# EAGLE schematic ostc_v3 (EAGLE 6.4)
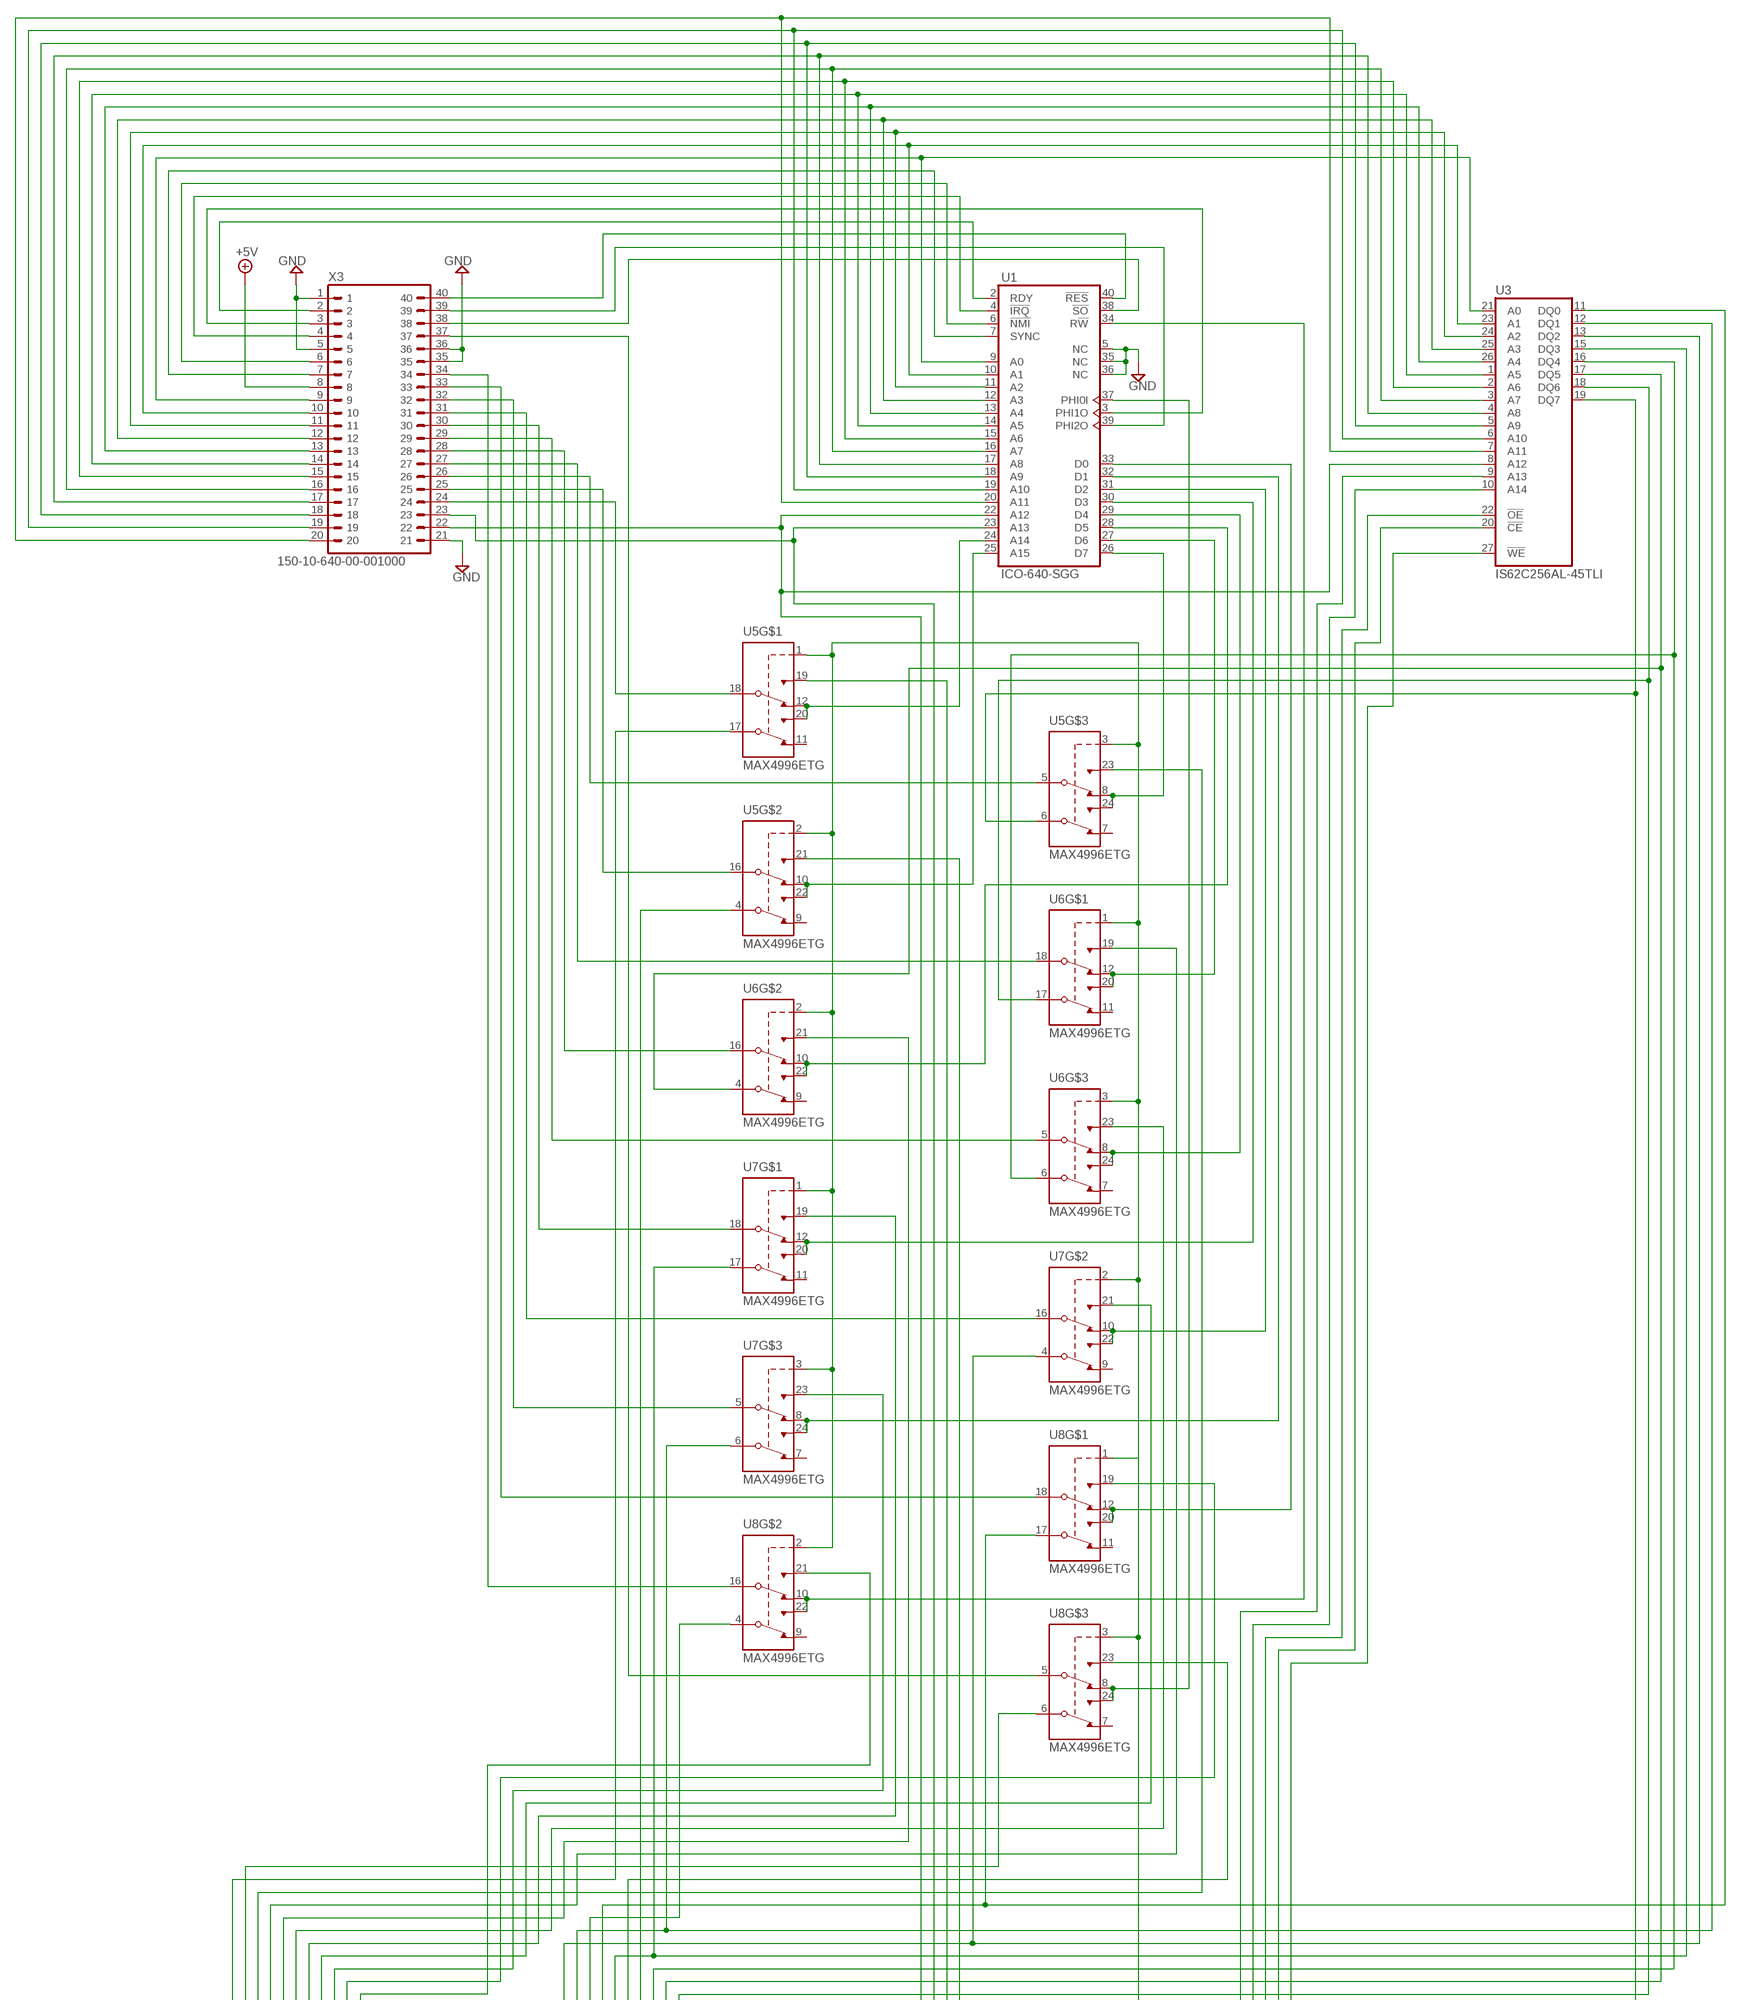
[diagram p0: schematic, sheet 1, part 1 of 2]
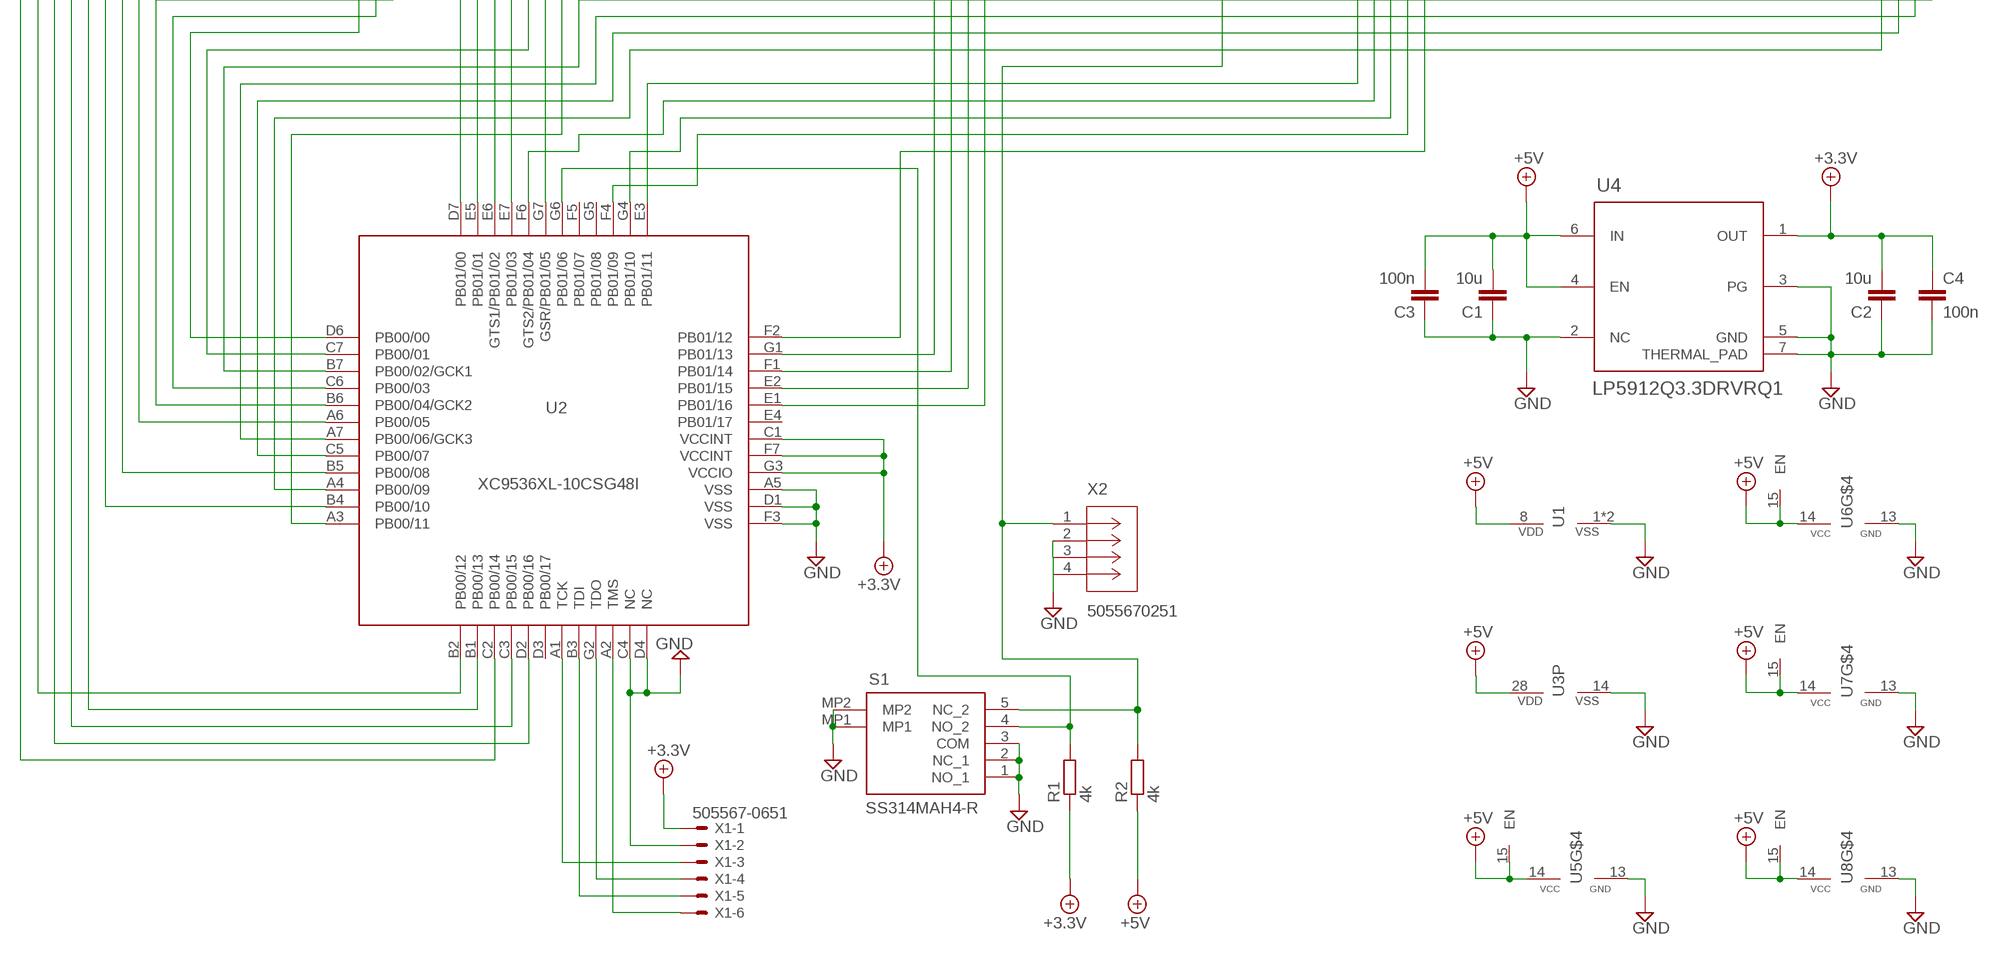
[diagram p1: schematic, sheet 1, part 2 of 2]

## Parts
C1  10u  C-EUC1206K  [C1206K]
C2  10u  C-EUC1206K  [C1206K]
C3  100n  C-EUC1206K  [C1206K]
C4  100n  C-EUC1206K  [C1206K]
R1  4k  R-EU_R0805  [R0805]
R2  4k  R-EU_R0805  [R0805]
S1  SS314MAH4-R  [SS314MAH4R]
U1  ICO-640-SGG  6502  [DIL40_LOWPROFILE]
U2  XC9536XL-10CSG48I  CX9536_CS48  [CSBGA48]
U3  IS62C256AL-45TLI  CY62256LL-ZC  [TSOP1-28]
U4  LP5912Q3.3DRVRQ1  LP5912-3.0DRVT  [DRV0006A-IPC_A]
U5  MAX4996ETG  [TQFN24]
U6  MAX4996ETG  [TQFN24]
U7  MAX4996ETG  [TQFN24]
U8  MAX4996ETG  [TQFN24]
X1  505567-0651  53261-06  [53261-06]
X2  5055670251  [CON_5055670251]
X3  150-10-640-00-001000  DIL40  [DIL40]

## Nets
+3.3V: C2.2 C4.1 R1.1 U2.C1(VCCINT) U2.F7(VCCINT) U2.G3(VCCIO) U4.1(OUT) X1.1
+5V: C1.2 C3.2 R2.1 U1.8(VDD) U3.28(VDD) U4.4(EN) U4.6(IN) U5.14(VCC) U5.15(EN) U6.14(VCC) U6.15(EN) U7.14(VCC) U7.15(EN) U8.14(VCC) U8.15(EN) X3.8
GND: C1.1 C2.1 C3.1 C4.2 S1.1(NO_1) S1.2(NC_1) S1.3(COM) S1.MP1 S1.MP2 U1.1(VSS) U1.5(NC) U1.21(VSS) U1.35(NC) U1.36(NC) U2.A5(VSS) U2.C4(NC) U2.D1(VSS) U2.D4(NC) U2.F3(VSS) U3.14(VSS) U4.2(NC) U4.3(PG) U4.5(GND) U4.7(THERMAL_PAD) U5.13(GND) U6.13(GND) U7.13(GND) U8.13(GND) X1.2 X2.2 X2.3 X2.4 X3.1 X3.5 X3.21 X3.35 X3.36
N$1: U1.2(RDY) X3.2
N$2: U1.3(PHI1O) X3.3
N$3: U1.4(!IRQ) X3.4
N$4: U1.6(!NMI) X3.6
N$5: U1.7(SYNC) X3.7
N$6: U1.9(A0) U3.21(A0) X3.9
N$7: U1.10(A1) U3.23(A1) X3.10
N$8: U1.11(A2) U3.24(A2) X3.11
N$9: U1.12(A3) U3.25(A3) X3.12
N$10: U1.13(A4) U3.26(A4) X3.13
N$11: U1.14(A5) U3.1(A5) X3.14
N$12: U1.15(A6) U3.2(A6) X3.15
N$13: U1.16(A7) U3.3(A7) X3.16
N$14: U1.17(A8) U3.4(A8) X3.17
N$15: U1.18(A9) U3.5(A9) X3.18
N$16: U1.19(A10) U3.6(A10) X3.19
N$17: U1.20(A11) U3.7(A11) X3.20
N$18: U2.E2(PB01/15) U5.19(NO1)
N$19: U1.22(A12) U2.G1(PB01/13) U3.8(A12) X3.22
N$20: U1.23(A13) U2.F1(PB01/14) X3.23
N$21: U2.E1(PB01/16) U5.21(NO1)
N$22: U2.D2(PB00/16) U5.23(NO1)
N$23: U2.C3(PB00/15) U6.19(NO1)
N$24: U2.B1(PB00/13) U6.21(NO1)
N$25: U2.B4(PB00/10) U6.23(NO1)
N$26: U2.B5(PB00/08) U7.19(NO1)
N$27: U2.A6(PB00/05) U7.21(NO1)
N$28: U2.B6(PB00/04/GCK2) U7.23(NO1)
N$29: U2.C6(PB00/03) U8.19(NO1)
N$30: U2.D6(PB00/00) U8.21(NO1)
N$31: U8.5(COM1) X3.37
N$32: U1.38(!SO) X3.38
N$33: U1.39(PHI2O) X3.39
N$34: U1.40(!RES) X3.40
N$35: U2.B2(PB00/12) U8.6(COM2)
N$36: U2.E6(GTS1/PB01/02) U8.4(COM2)
N$37: U2.E7(PB01/03) U3.11(DQ0) U8.17(COM2)
N$38: U2.E5(PB01/01) U3.12(DQ1) U7.6(COM2)
N$39: U2.D7(PB01/00) U3.13(DQ2) U7.4(COM2)
N$40: U2.C7(PB00/01) U3.15(DQ3) U7.17(COM2)
N$41: U2.B7(PB00/02/GCK1) U3.16(DQ4) U6.6(COM2)
N$42: U2.A7(PB00/06/GCK3) U3.17(DQ5) U6.4(COM2)
N$43: U2.C5(PB00/07) U3.18(DQ6) U6.17(COM2)
N$44: U2.A4(PB00/09) U3.19(DQ7) U5.6(COM2)
N$45: R1.2 S1.4(NO_2) U2.G6(PB01/06)
N$46: U1.24(A14) U5.12(NC1) U5.20(NO2)
N$47: U1.26(D7) U5.8(NC1) U5.24(NO2)
N$48: U5.16(COM1) X3.25
N$49: U1.25(A15) U5.10(NC1) U5.22(NO2)
N$50: U5.5(COM1) X3.26
N$51: R2.2 S1.5(NC_2) U5.1(CB) U5.2(CB) U5.3(CB) U6.1(CB) U6.2(CB) U6.3(CB) U7.1(CB) U7.2(CB) U7.3(CB) U8.1(CB) U8.2(CB) U8.3(CB) X2.1
N$52: U6.18(COM1) X3.27
N$53: U2.A3(PB00/11) U5.4(COM2)
N$54: U2.C2(PB00/14) U5.17(COM2)
N$55: U2.A2(TMS) X1.6
N$56: U2.B3(TDI) X1.5
N$57: U2.G2(TDO) X1.4
N$58: U2.A1(TCK) X1.3
N$59: U1.27(D6) U6.12(NC1) U6.20(NO2)
N$60: U5.18(COM1) X3.24
N$61: U6.16(COM1) X3.28
N$62: U1.28(D5) U6.10(NC1) U6.22(NO2)
N$63: U7.16(COM1) X3.31
N$64: U1.29(D4) U6.8(NC1) U6.24(NO2)
N$65: U6.5(COM1) X3.29
N$66: U7.18(COM1) X3.30
N$67: U1.30(D3) U7.12(NC1) U7.20(NO2)
N$68: U1.31(D2) U7.10(NC1) U7.22(NO2)
N$69: U7.5(COM1) X3.32
N$70: U1.32(D1) U7.8(NC1) U7.24(NO2)
N$71: U1.33(D0) U8.12(NC1) U8.20(NO2)
N$72: U8.18(COM1) X3.33
N$73: U8.16(COM1) X3.34
N$74: U1.34(R!W) U8.10(NC1) U8.22(NO2)
N$75: U1.37(PHI0I) U8.8(NC1) U8.24(NO2)
N$76: U2.G7(GSR/PB01/05) U8.23(NO1)
N$77: U2.E3(PB01/11) U3.9(A13)
N$78: U2.F6(GTS2/PB01/04) U3.10(A14)
N$79: U2.G4(PB01/10) U3.22(!OE)
N$80: U2.F4(PB01/09) U3.20(!CE)
N$81: U2.F2(PB01/12) U3.27(!WE)
Unconnected: U2.D3(PB00/17) U2.E4(PB01/17) U2.F5(PB01/07) U2.G5(PB01/08) U5.7(NC2) U5.9(NC2) U5.11(NC2) U6.7(NC2) U6.9(NC2) U6.11(NC2) U7.7(NC2) U7.9(NC2) U7.11(NC2) U8.7(NC2) U8.9(NC2) U8.11(NC2)

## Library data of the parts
C1-C4 = resistor:C-EU: CAPACITOR, European symbol
R1 R2 = resistor:R-EU_: RESISTOR, European symbol
S1 = SS314MAH4-R:SS314MAH4-R: Slide Switches ON-ON-ON .4VA SMT 2MM X 2MM SPACING Source: Datasheet; DESCRIPTION: Slide Switches ON-ON-ON .4VA SMT 2MM X 2MM SPACING; HEIGHT: 1.4mm; MANUFACTURER_NAME: NKK Switches; MANUFACTURER_PART_NUMBER: SS314MAH4-R; MOUSER_PART_NUMBER: 633-SS314MAH4-R; MOUSER_PRICE-STOCK: https://www.mouser.co.uk/ProductDetail/NKK-Switches/SS314MAH4-R?qs=ICf24S48Y%2FuhNriUiZqPNA%3D%3D
U1 = 6502:6502: R6502 by Rockwell
U2 = xilinx-xc9:CX9536_CS48
U3 = memory-sram:CY62256LL-?*: 256K (32K x 8) CMOS-Static RAM Source: http://download.cypress.com.edgesuite.net/design_resources/datasheets/contents/cy62256_8.pdf
U4 = texas:LP5912-3.0DRVT; COPYRIGHT: Copyright (C) 2024 Ultra Librarian. All rights reserved.; MANUFACTURER_PART_NUMBER: LP5912-3.0DRVT; MFR_NAME: Texas Instruments; REFDES: RefDes; TYPE: TYPE
U5-U8 = maxim:MAX4996ETG*: Triple DPDT, Low Capacitance Data Switches * No exposed pad Source: https://www.analog.com/media/en/technical-documentation/data-sheets/max4996-max4996l.pdf; MPN: MAX4996ETG+; OC_MOUSER: 700-MAX4996ETG
X1 = con-molex:53?-06: CONNECTOR wire to board 1.25 mm (.049 inch) pitch header; OC_FARNELL: 1125375; OC_NEWARK: unknown
X2 = con-molex:5055670251; COPYRIGHT: Copyright (C) 2024 Ultra Librarian. All rights reserved.; MANUFACTURER_PART_NUMBER: 5055670251; MFR_NAME: Molex Connector Corporation
X3 = DIL-header:DIL40: DIL Header 40-pin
